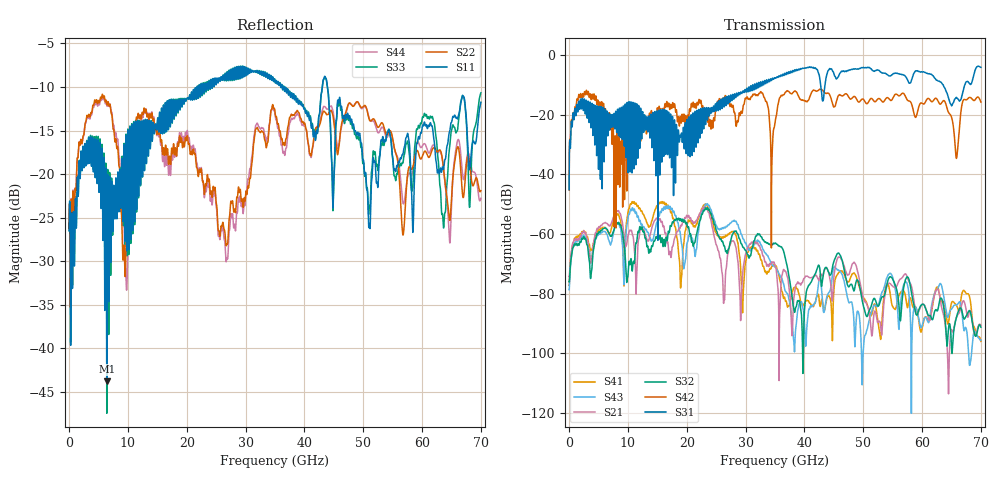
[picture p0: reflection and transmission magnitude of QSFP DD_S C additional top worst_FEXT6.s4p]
! AWR Design Environment (8415) Thu Dec 20 17:03:43 2018
! Document = 'CHANNEL TEST'
! nPorts: 4, nXvals: 7001
# HZ S DB R 50
!Freq DBS11 AngS11 DBS12 AngS12 DBS13 AngS13 DBS14 AngS14
!	DBS21 AngS21 DBS22 AngS22 DBS23 AngS23 DBS24 AngS24
!	DBS31 AngS31 DBS32 AngS32 DBS33 AngS33 DBS34 AngS34
!	DBS41 AngS41 DBS42 AngS42 DBS43 AngS43 DBS44 AngS44
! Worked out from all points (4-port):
!   7000 points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, 10 MHz to 70 GHz, reference 50 ohm
!   strongest paths, dB at 10 MHz, 17.51 GHz, 35.01 GHz, 52.51 GHz, 70 GHz:
!     S31: -45.1, -23.1, -7.6, -5.0, -4.0
!     S42: -45.2, -17.2, -22.6, -14.6, -15.7
!     S32: -76.1, -56.2, -63.1, -84.2, -91.3
!     S21: -74.3, -64.6, -70.7, -89.7, -90.7
!     S43: -78.8, -51.5, -71.1, -84.1, -95.7
!     S41: -77.3, -53.5, -70.5, -89.5, -96.1
!   lowest |S11| = -43.8 dB at 6.41 GHz (marker M1), VSWR 1.01, Z = 50.5 - j0.428 ohm
!   |S11| at or under -10 dB: start of sweep to 21.78 GHz; 36.52 GHz to 43.04 GHz (6.515 GHz wide, 16.4 % of centre); 43.91 GHz to end of sweep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
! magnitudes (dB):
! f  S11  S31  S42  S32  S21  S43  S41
! 10 MHz  -26.5  -45.1  -45.2  -76.1  -74.3  -78.8  -77.3
! 1.66 GHz  -19.6  -15.4  -13.2  -63.7  -62.0  -62.3  -61.0
! 6.41 GHz  -43.8  -18.7  -22.2  -58.4  -56.5  -60.0  -58.5
! 9.67 GHz  -15.6  -23.6  -27.6  -71.9  -64.1  -60.4  -58.2
! 23.45 GHz  -9.5  -19.6  -20.8  -51.2  -51.4  -49.9  -50.3
! 26.28 GHz  -8.8  -16.5  -14.4  -63.9  -83.1  -58.0  -60.9
! 70 GHz  -11.8  -4.0  -15.7  -91.3  -90.7  -95.7  -96.1
